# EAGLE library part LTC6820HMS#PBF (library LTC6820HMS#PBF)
Interface - Specialized isoSPI Iso Communications Int Source: Datasheet
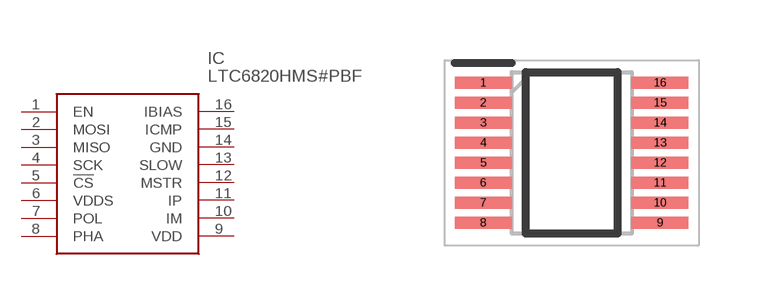
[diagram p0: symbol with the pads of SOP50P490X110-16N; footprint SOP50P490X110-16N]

Designator prefix IC

## LTC6820HMS#PBF (Description: Interface - Specialized isoSPI Iso Communications Int; Height: 1.1mm; Manufacturer_Name: Analog Devices; Manufacturer_Part_Number: LTC6820HMS#PBF; Mouser_Part_Number: 584-LTC6820HMS#PBF; Mouser_Price-Stock: https://www.mouser.co.uk/ProductDetail/Analog-Devices/LTC6820HMSPBF?qs=hVkxg5c3xu%252BAhS55eUb%252BEQ%3D%3D)  [SOP50P490X110-16N]
1  EN
2  MOSI
3  MISO
4  SCK
5  !CS
6  VDDS
7  POL
8  PHA
9  VDD
10  IM
11  IP
12  MSTR
13  SLOW
14  GND
15  ICMP
16  IBIAS

## Footprint SOP50P490X110-16N (pad centres in mm)
msop-16
smd 1.425 x 0.3: 1 -2.212,1.75; 2 -2.212,1.25; 3 -2.212,0.75; 4 -2.212,0.25; 5 -2.212,-0.25; 6 -2.212,-0.75; 7 -2.212,-1.25; 8 -2.212,-1.75; 9 2.212,-1.75; 10 2.212,-1.25; 11 2.212,-0.75; 12 2.212,-0.25; 13 2.212,0.25; 14 2.212,0.75; 15 2.212,1.25; 16 2.212,1.75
